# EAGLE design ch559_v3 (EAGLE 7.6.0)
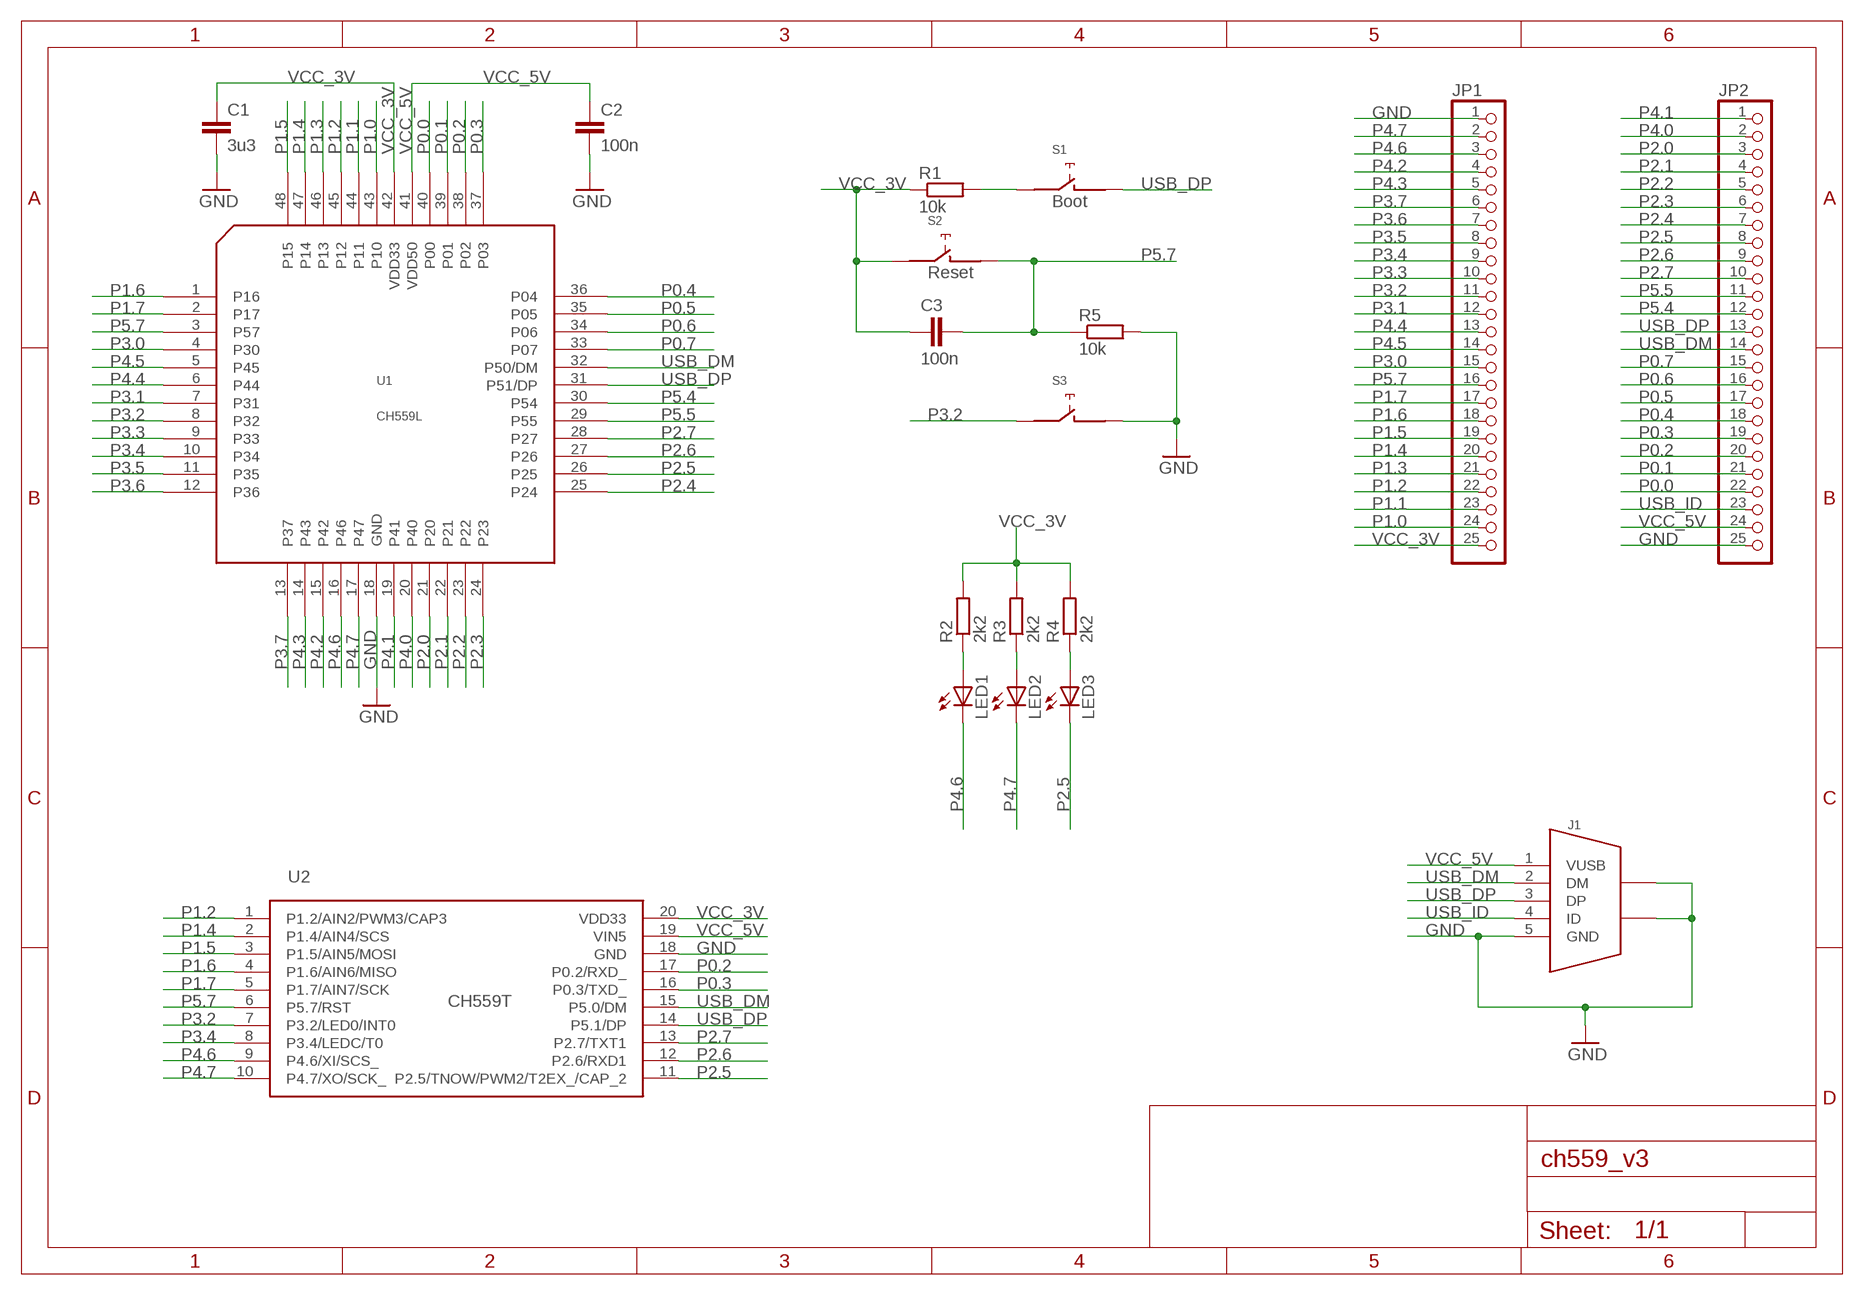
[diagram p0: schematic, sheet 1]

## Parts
C1  3u3  C-EUC0805  [C0805]
C2  100n  C-EUC0805  [C0805]
C3  100n  C-EUC0805  [C0805]
J1  MIC_USB_BBU  [MICRO_USB_B]
JP1  PINHD25  [1X25]
JP2  PINHD25  [1X25]
LED1  LEDSML0805  [SML0805]
LED2  LEDSML0805  [SML0805]
LED3  LEDSML0805  [SML0805]
R1  10k  R-EU_R0603  [R0603]
R2  2k2  R-EU_R0603  [R0603]
R3  2k2  R-EU_R0603  [R0603]
R4  2k2  R-EU_R0603  [R0603]
R5  10k  R-EU_R0603  [R0603]
S1  KMR_231_G_LFS  [KMR_231]
S2  KMR_231_G_LFS  [KMR_231]
S3  KMR_231_G_LFS  [KMR_231]
U1  CH559L  [LQFP48]
U2  CH559T  [SSOP20]

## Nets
GND: C1.2 C2.2 J1.5(GND) J1.P3(SHIELD) J1.P4(SHIELD) JP1.1 JP2.25 R5.2 S3.P$3 S3.P$4 U1.18(GND) U2.18(GND)
N$2: LED1.A R2.1
N$30: R1.2 S1.P$1 S1.P$2
N$43: LED2.A R3.1
N$44: LED3.A R4.1
P0.0: JP2.22 U1.40(P00)
P0.1: JP2.21 U1.39(P01)
P0.2: JP2.20 U1.38(P02) U2.17(P0.2/RXD_)
P0.3: JP2.19 U1.37(P03) U2.16(P0.3/TXD_)
P0.4: JP2.18 U1.36(P04)
P0.5: JP2.17 U1.35(P05)
P0.6: JP2.16 U1.34(P06)
P0.7: JP2.15 U1.33(P07)
P1.0: JP1.24 U1.43(P10)
P1.1: JP1.23 U1.44(P11)
P1.2: JP1.22 U1.45(P12) U2.1(P1.2/AIN2/PWM3/CAP3)
P1.3: JP1.21 U1.46(P13)
P1.4: JP1.20 U1.47(P14) U2.2(P1.4/AIN4/SCS)
P1.5: JP1.19 U1.48(P15) U2.3(P1.5/AIN5/MOSI)
P1.6: JP1.18 U1.1(P16) U2.4(P1.6/AIN6/MISO)
P1.7: JP1.17 U1.2(P17) U2.5(P1.7/AIN7/SCK)
P2.0: JP2.3 U1.21(P20)
P2.1: JP2.4 U1.22(P21)
P2.2: JP2.5 U1.23(P22)
P2.3: JP2.6 U1.24(P23)
P2.4: JP2.7 U1.25(P24)
P2.5: JP2.8 LED3.C U1.26(P25) U2.11(P2.5/TNOW/PWM2/T2EX_/CAP_2)
P2.6: JP2.9 U1.27(P26) U2.12(P2.6/RXD1)
P2.7: JP2.10 U1.28(P27) U2.13(P2.7/TXT1)
P3.0: JP1.15 U1.4(P30)
P3.1: JP1.12 U1.7(P31)
P3.2: JP1.11 S3.P$1 S3.P$2 U1.8(P32) U2.7(P3.2/LED0/INT0)
P3.3: JP1.10 U1.9(P33)
P3.4: JP1.9 U1.10(P34) U2.8(P3.4/LEDC/T0)
P3.5: JP1.8 U1.11(P35)
P3.6: JP1.7 U1.12(P36)
P3.7: JP1.6 U1.13(P37)
P4.0: JP2.2 U1.20(P40)
P4.1: JP2.1 U1.19(P41)
P4.2: JP1.4 U1.15(P42)
P4.3: JP1.5 U1.14(P43)
P4.4: JP1.13 U1.6(P44)
P4.5: JP1.14 U1.5(P45)
P4.6: JP1.3 LED1.C U1.16(P46) U2.9(P4.6/XI/SCS_)
P4.7: JP1.2 LED2.C U1.17(P47) U2.10(P4.7/XO/SCK_)
P5.4: JP2.12 U1.30(P54)
P5.5: JP2.11 U1.29(P55)
P5.7: C3.2 JP1.16 R5.1 S2.P$3 S2.P$4 U1.3(P57) U2.6(P5.7/RST)
USB_DM: J1.2(DM) JP2.14 U1.32(P50/DM) U2.15(P5.0/DM)
USB_DP: J1.3(DP) JP2.13 S1.P$3 S1.P$4 U1.31(P51/DP) U2.14(P5.1/DP)
USB_ID: J1.4(ID) JP2.23
VCC_3V: C1.1 C3.1 JP1.25 R1.1 R2.2 R3.2 R4.2 S2.P$1 S2.P$2 U1.42(VDD33) U2.20(VDD33)
VCC_5V: C2.1 J1.1(VUSB) JP2.24 U1.41(VDD50) U2.19(VIN5)

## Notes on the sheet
- Boot
- Reset

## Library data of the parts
C1-C3 = rcl:C-EU: CAPACITOR, European symbol
J1 = tzlib:MIC_USB_BBU
JP1 JP2 = tzlib:PINHD25
LED1-LED3 = led:LED: LED
R1-R5 = rcl:R-EU_: RESISTOR, European symbol
S1-S3 = tzlib:KMR_231_G_LFS
U1 = tzlib:CH559L
U2 = tzlib:CH559T

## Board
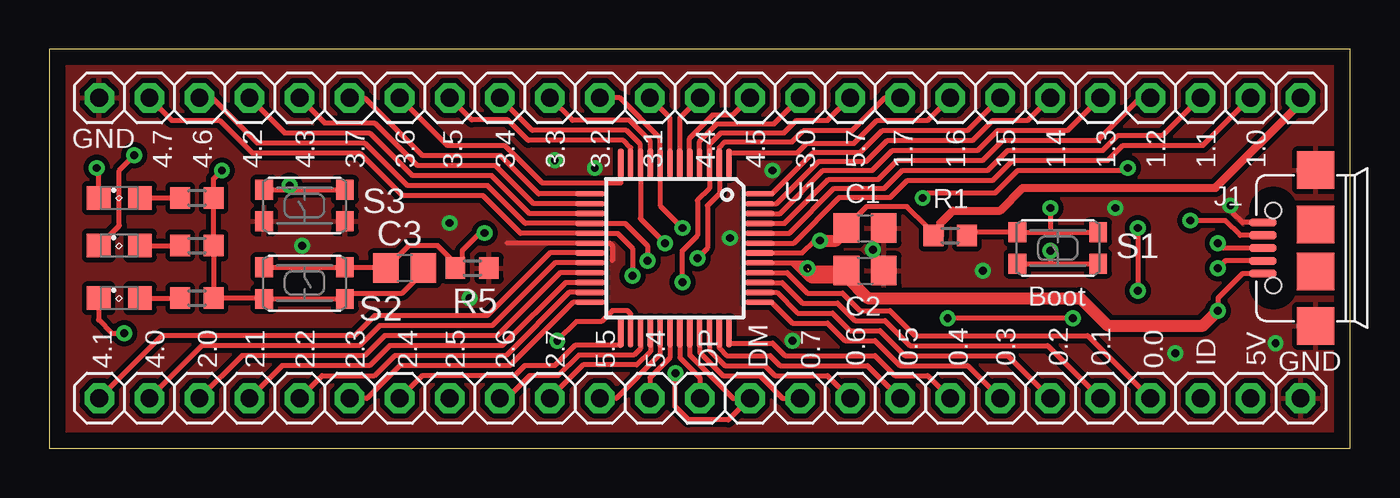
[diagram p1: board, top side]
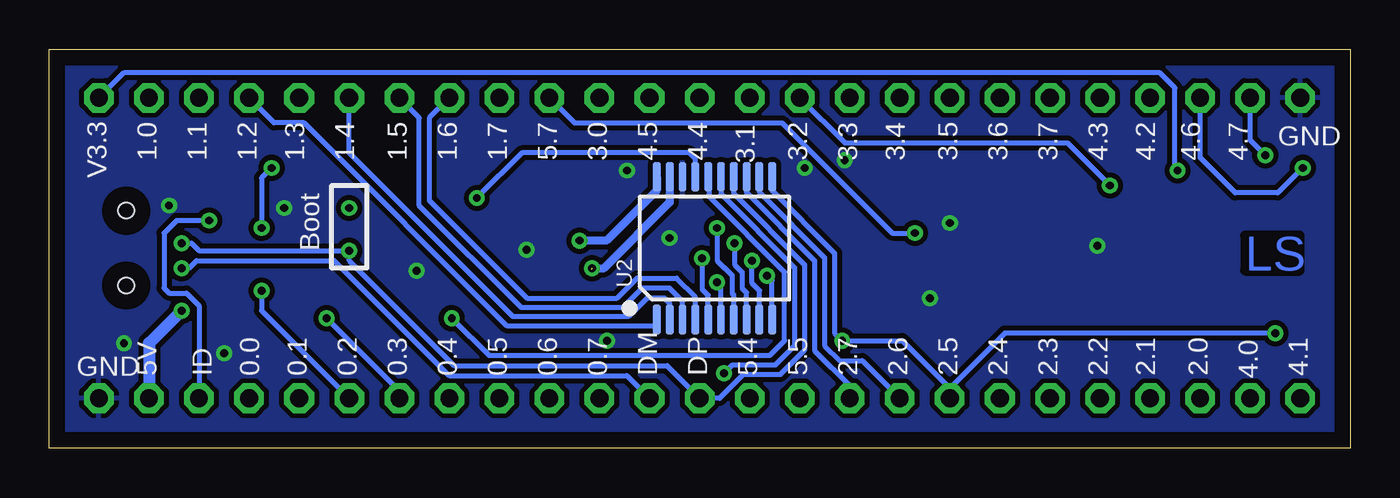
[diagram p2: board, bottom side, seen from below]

Size 66.02 x 20.24 mm. Coordinates in mm from the lower left corner, seen from the top.
Outline: 0,0 66.02,0 66.02,20.24 0,20.24 0,0
Copper layers (1*16): Top 0.035mm / dielectric 1.5mm / Bottom 0.035mm
Design rules "default *": minimum track width 8mil, minimum drill 0.4mm, track to track 0.16mm, track to pad 0.16mm, pad to pad 0.2mm, via to via 0.2mm, smd to smd 0.2mm, copper to edge 32mil, drill to drill 8mil, minimum pad ring 10mil, minimum via ring 8mil, stop-mask expansion 4mil, vias tented up to drill 0mil, thermal gap 10mil

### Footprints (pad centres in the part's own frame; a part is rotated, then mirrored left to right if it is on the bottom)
C0805 = smd 1.3 x 1.5: 1 -0.95,0; 2 0.95,0
MICRO_USB_B = smd 0.4 x 1.4: 1 -1.3,2.675; 2 -0.65,2.675; 3 0,2.675; 4 0.65,2.675; 5 1.3,2.675 | smd 1.9 x 1.9: P1 -1.2,0; P2 1.2,0; P3 3.95,0; P4 -3.95,0 | hole 0.8: -1.9,2.15; 1.9,2.15
1X25 = drill 0.9 pad 1.5 octagon: 1 -29.21,0; 2 -26.67,0; 3 -24.13,0; 4 -21.59,0; 5 -19.05,0; 6 -16.51,0; 7 -13.97,0; 8 -11.43,0; 9 -8.89,0; 10 -6.35,0; 11 -3.81,0; 12 -1.27,0; 13 1.27,0; 14 3.81,0; 15 6.35,0; 16 8.89,0; 17 11.43,0; 18 13.97,0; 19 16.51,0; 20 19.05,0; 21 21.59,0; 22 24.13,0; 23 26.67,0; 24 29.21,0; 25 31.75,0
SML0805 = smd 1.2 x 1.2: A 1.05,0; C -1.05,0
R0603 = smd 1 x 1.1: 1 -0.85,0; 2 0.85,0
KMR_231 = smd 0.9 x 1: P$1 -2.05,0.8; P$2 2.05,0.8; P$3 -2.05,-0.8; P$4 2.05,-0.8
LQFP48 = smd 1.5 x 0.3: 1 -4.3,2.75; 2 -4.3,2.25; 3 -4.3,1.75; 4 -4.3,1.25; 5 -4.3,0.75; 6 -4.3,0.25; 7 -4.3,-0.25; 8 -4.3,-0.75; 9 -4.3,-1.25; 10 -4.3,-1.75; 11 -4.3,-2.25; 12 -4.3,-2.75; 25 4.3,-2.75; 26 4.3,-2.25; 27 4.3,-1.75; 28 4.3,-1.25; 29 4.3,-0.75; 30 4.3,-0.25; 31 4.3,0.25; 32 4.3,0.75; 33 4.3,1.25; 34 4.3,1.75; 35 4.3,2.25; 36 4.3,2.75 | smd 0.3 x 1.5: 13 -2.75,-4.3; 14 -2.25,-4.3; 15 -1.75,-4.3; 16 -1.25,-4.3; 17 -0.75,-4.3; 18 -0.25,-4.3; 19 0.25,-4.3; 20 0.75,-4.3; 21 1.25,-4.3; 22 1.75,-4.3; 23 2.25,-4.3; 24 2.75,-4.3; 37 2.75,4.3; 38 2.25,4.3; 39 1.75,4.3; 40 1.25,4.3; 41 0.75,4.3; 42 0.25,4.3; 43 -0.25,4.3; 44 -0.75,4.3; 45 -1.25,4.3; 46 -1.75,4.3; 47 -2.25,4.3; 48 -2.75,4.3
SSOP20 = smd 0.4 x 1.5: 1 -2.925,-3.625; 2 -2.275,-3.625; 3 -1.625,-3.625; 4 -0.975,-3.625; 5 -0.325,-3.625; 6 0.325,-3.625; 7 0.975,-3.625; 8 1.625,-3.625; 9 2.275,-3.625; 10 2.925,-3.625; 11 2.925,3.625; 12 2.275,3.625; 13 1.625,3.625; 14 0.975,3.625; 15 0.325,3.625; 16 -0.325,3.625; 17 -0.975,3.625; 18 -1.625,3.625; 19 -2.275,3.625; 20 -2.925,3.625

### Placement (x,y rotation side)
C1  41.4,11.18 0 top
C2  41.4,9.02 0 top
C3  18.03,9.14 180 top
J1  64.26,10.16 90 top
JP1  31.75,17.78 0 top
JP2  31.75,2.54 0 top
LED1  3.56,12.7 0 top
LED2  3.56,10.29 0 top
LED3  3.56,7.62 0 top
R1  45.72,10.79 0 top
R2  7.49,12.7 0 top
R3  7.49,10.29 0 top
R4  7.49,7.62 0 top
R5  21.46,9.14 0 top
S1  51.18,10.16 0 top
S2  12.95,8.38 180 top
S3  12.95,12.32 0 top
U1  31.75,10.16 270 top
U2  32.26,10.16 0 bottom

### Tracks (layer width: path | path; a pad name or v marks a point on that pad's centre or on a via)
GND  (via drill 0.4)
  Top 0.254: 27.44,10.41 27.43,10.41 | J1.5 60.55,11.46 60.07,11.94 | 27.44,10.41 23.24,10.41 | 27.44,10.41 28.45,10.41 28.57,10.29 28.57,9.53
  Top 0.813: J1.P4 64.26,6.1 | J1.P3 64.26,14.61
  other vias: 34.54,10.67 12.83,10.29 20.32,11.43 41.81,10.08 47.37,9.02 57.15,4.83 54.1,12.19 59.94,12.32 62.23,5.33 37.72,5.46 21.34,7.62 27.69,14.22 25.65,14.61 36.7,14.1
  pour Bottom (isolate 0.254): 0.51,20.07 65.79,20.07 65.79,0.13 0.51,0.13
  pour Top (isolate 0.254): 0.25,20.19 66.04,20.19 66.04,0 0.25,0
N$2
  Top 0.254: LED1.A R2.1
N$30  (via drill 0.4)
  Top 0.254: 50.8,10.96 S1.P$1 46.73,10.96 R1.2 | 50.8,10.96 S1.P$2 | v50.8,12.19 50.8,10.96
N$43
  Top 0.254: LED2.A R3.1
N$44
  Top 0.254: LED3.A R4.1
P0.0
  Top 0.254: U1.40 37.45,8.91 38.35,8 38.48,7.87 40.26,7.87 41.15,6.99 42.67,6.99 43.94,5.71 52.7,5.71 JP2.22
P0.1
  Top 0.254: U1.39 37.18,8.41 38.23,7.37 40.01,7.37 40.89,6.48 42.42,6.48 43.69,5.21 50.67,5.21 JP2.21
P0.2  (via drill 0.4)
  Top 0.254: U1.38 36.92,7.91 37.97,6.86 39.75,6.86 40.64,5.97 42.16,5.97 43.43,4.7 48.64,4.7 JP2.20 | v44.32,12.7 44.58,12.95 48.01,12.95 49.15,14.1 54.61,14.1 v54.74,14.22 | v55.25,11.18 v55.25,8
  Bottom 0.254: v54.74,14.22 55.25,13.72 v55.25,11.18 | JP2.20 55.25,6.99 v55.25,8 | U2.17 33.23,14.69 33.53,14.99 42.04,14.99 v44.32,12.7
P0.3  (via drill 0.4)
  Top 0.254: U1.37 36.66,7.41 37.72,6.35 39.5,6.35 40.39,5.46 41.91,5.46 43.18,4.19 46.61,4.19 JP2.19 | v51.94,6.6 v45.59,6.6
  Bottom 0.254: JP2.19 48.26,2.92 v51.94,6.6 | v45.59,6.6 43.69,4.7 29.46,4.7 28.7,5.46 28.7,8.94 32.51,12.75 32.51,13.71 U2.16
P0.4
  Top 0.254: U1.36 34.5,5.38 34.54,5.33 36.7,5.33 37.34,4.7 41.91,4.7 42.93,3.68 44.58,3.68 JP2.18
P0.5
  Top 0.254: U1.35 34,5.08 34.38,4.7 36.58,4.7 37.08,4.19 41.53,4.19 JP2.17
P0.6
  Top 0.254: JP2.16 39.5,3.68 36.83,3.68 36.32,4.19 34.29,4.19 33.5,4.98 U1.34
P0.7
  Top 0.254: U1.33 33,4.87 34.19,3.68 36.07,3.68 37.21,2.54 JP2.15
P1.0
  Top 0.254: U1.43 37.78,10.41 40.09,12.72 42.7,12.72 43.56,13.59 47.88,13.59 48.89,14.61 53.72,14.61 54.48,15.37 58.55,15.37 JP1.24
P1.1
  Top 0.254: U1.44 37.55,10.91 39.83,13.18 42.39,13.18 43.31,14.1 47.62,14.1 48.64,15.11 53.47,15.11 54.23,15.88 56.52,15.88 JP1.23
P1.2
  Top 0.254: U1.45 37.32,11.41 39.55,13.64 42.09,13.64 43.05,14.61 47.37,14.61 48.39,15.62 53.21,15.62 55.37,17.78 JP1.22
  Bottom 0.254: JP1.22 54.61,16.51 53.09,16.51 42.78,6.2 35.35,6.2 35.18,6.37 U2.1
P1.3
  Top 0.254: U1.46 37.08,11.91 39.27,14.1 41.78,14.1 42.8,15.11 47.12,15.11 48.13,16.13 51.69,16.13 JP1.21
P1.4
  Top 0.254: U1.47 36.91,12.41 39.05,14.55 41.48,14.55 42.55,15.62 46.86,15.62 47.88,16.64 49.66,16.64 JP1.20
  Bottom 0.254: JP1.20 50.8,14.99 42.49,6.68 36.63,6.68 35.69,7.62 34.8,7.62 34.53,7.36 U2.2
P1.5
  Top 0.254: JP1.19 46.61,16.13 42.29,16.13 41.17,15.01 38.79,15.01 36.68,12.91 U1.48
  Bottom 0.254: JP1.19 47.24,16.76 47.24,12.32 42.06,7.14 36.93,7.14 35.94,8.13 34.54,8.13 33.88,7.47 U2.3
P1.6
  Top 0.254: JP1.18 44.58,16.64 42.01,16.64 40.84,15.47 38.46,15.47 37.97,14.99 34.52,14.99 34.5,14.97 U1.1
  Bottom 0.254: JP1.18 46.74,16.76 46.74,12.57 41.78,7.62 37.21,7.62 36.2,8.64 34.19,8.64 33.23,7.68 U2.4
P1.7  (via drill 0.4)
  Top 0.254: v32.89,9.65 33.4,10.16 33.4,12.32 34,12.92 U1.2 34,15.25 34.29,15.54 37.69,15.54 38.25,16.1 40.74,16.1 42.42,17.78 JP1.17
  Bottom 0.254: U2.5 32.58,7.77 32.89,8.08 v32.89,9.65
P2.0
  Top 0.254: U1.21 25.93,8.91 22.73,5.71 17.02,5.71 16,4.7 9.78,4.7 JP2.3
P2.1
  Top 0.254: U1.22 26.19,8.41 22.99,5.21 17.27,5.21 16.26,4.19 11.81,4.19 JP2.4
P2.2
  Top 0.254: U1.23 26.39,7.91 23.18,4.7 17.53,4.7 16.51,3.68 13.84,3.68 JP2.5
P2.3
  Top 0.254: U1.24 26.59,7.41 23.37,4.19 17.78,4.19 16.13,2.54 JP2.6
P2.4
  Top 0.254: U1.25 29,5.25 28.97,5.23 26.69,5.23 25.65,4.19 24.13,4.19 23.62,3.68 18.92,3.68 JP2.7
P2.5  (via drill 0.4)
  Top 0.254: U1.26 29.5,6.82 29.34,6.99 28.57,6.99 28.02,6.43 26.75,6.43 v25.78,5.46 | LED3.C 2.51,6.51 3.18,5.84 v3.81,5.84
  Bottom 0.254: 20.32,3.05 22.73,5.46 v25.78,5.46 26.16,5.84 26.16,9.91 29.34,13.08 U2.11 | 20.32,3.05 JP2.8 | v3.81,5.84 17.53,5.84 20.32,3.05
P2.6
  Top 0.254: U1.27 30,5.06 29.67,4.72 26.87,4.72 25.83,3.68 24.38,3.68 23.24,2.54 JP2.9
  Bottom 0.254: JP2.9 24.77,4.45 25.91,4.45 26.67,5.21 26.67,9.68 29.97,12.98 U2.12
P2.7
  Top 0.254: U1.28 30.5,4.91 29.82,4.23 27.09,4.23 JP2.10
  Bottom 0.254: JP2.10 25.4,3.17 27.18,4.95 27.18,9.53 30.63,12.98 U2.13
P3.0
  Top 0.254: U1.4 33,15.58 33.88,16.46 36.78,16.46 JP1.15
P3.1
  Top 0.254: U1.7 31.5,16.76 JP1.12
P3.2  (via drill 0.4)
  Top 0.254: JP1.11 28.96,17.78 31,15.74 U1.8 31,12.31 v32.13,11.18 | v12.19,13.34 12.15,13.34 12.19,13.12 | S3.P$1 12.19,13.12 | 12.19,13.12 S3.P$2
  Bottom 0.254: 12.19,13.59 v12.19,13.34 14.35,15.49 25.65,15.49 JP1.11 | v32.13,11.18 32.13,9.53 31.75,9.14 31.75,9.17 31.37,8.79 31.37,7.87 31.29,7.8 31.29,7.77 31.28,7.76 U2.7
P3.3
  Top 0.254: U1.9 30.5,15.58 29.44,16.64 26.54,16.64 JP1.10
P3.4  (via drill 0.4)
  Top 0.254: JP1.9 24.51,16.13 29.29,16.13 30,15.41 U1.10 30,11.66 v31.24,10.41
  Bottom 0.254: v31.24,10.41 31.24,9.32 30.86,8.94 30.86,8.13 30.63,7.9 U2.8 30.61,6.56
P3.5
  Top 0.254: U1.11 29.5,15.25 29.13,15.62 24.31,15.62 23.27,16.66 21.44,16.66 JP1.8
P3.6
  Top 0.254: 29,14.94 U1.12 29,13.46 25.02,13.46 23.11,15.37 20.19,15.37 JP1.7
P3.7
  Top 0.254: U1.13 24.83,12.91 22.88,14.86 18.92,14.86 16,17.78 JP1.6
P4.0
  Top 0.254: U1.20 25.67,9.41 22.48,6.22 16.76,6.22 15.75,5.21 7.75,5.21 JP2.2
P4.1
  Top 0.254: U1.19 25.4,9.91 22.23,6.73 16.51,6.73 15.49,5.71 5.71,5.71 JP2.1
P4.2
  Top 0.254: U1.15 24.36,11.91 22.43,13.84 18.41,13.84 16.26,16 11.94,16 JP1.4
P4.3
  Top 0.254: U1.14 24.57,12.41 22.63,14.35 18.67,14.35 16.51,16.51 13.97,16.51 JP1.5
P4.4
  Top 0.254: U1.6 32,16.76 JP1.13
P4.5
  Top 0.254: U1.5 32.5,15.74 33.68,16.92 34.7,16.92 JP1.14
P4.6  (via drill 0.4)
  Top 0.254: JP1.3 8.25,17.78 10.54,15.49 16,15.49 18.16,13.34 22.23,13.34 24.15,11.41 U1.16 29.23,11.41 30.35,10.29 v30.35,9.53 | LED1.C 2.51,14.13 v2.41,14.22
  Bottom 0.254: v2.41,14.22 3.68,12.95 5.84,12.95 7.62,14.73 JP1.3 | U2.9 29.98,7.25 29.97,7.26 29.97,8 30.35,8.38 v30.35,9.53
P4.7  (via drill 0.4)
  Top 0.254: JP1.2 6.22,16.64 8.64,16.64 10.29,14.99 15.75,14.99 17.91,12.83 22,12.83 23.91,10.91 U1.17 28.84,10.91 29.59,10.16 v29.59,8.76 | LED2.C 2.54,10.29 3.56,11.3 3.56,14.1 v4.32,14.86
  Bottom 0.254: v4.32,14.86 5.08,15.62 JP1.2 | U2.10 29.33,8.51 v29.59,8.76
P5.4
  Top 0.254: U1.30 31.5,4.6 30.48,3.58 JP2.12
P5.5
  Top 0.254: U1.29 31,4.76 28.78,2.54 JP2.11 28.3,2.54
P5.7  (via drill 0.4)
  Top 0.254: v32.13,8.43 32.13,10.03 32.89,10.79 32.89,12.57 33.5,13.18 U1.3 33.5,15.41 34.09,16 37.29,16 37.92,16.64 39.5,16.64 JP1.16 | S2.P$4 S2.P$3 17.08,9.18 C3.2 18.23,10.29 19.71,10.29 20.34,9.65 20.34,9.41 R5.1 | R5.1 20.61,9.36 | R5.1 20.95,9.49 20.95,10.03 21.84,10.92 v22.1,10.92
  Bottom 0.254: JP1.16 39.37,16.51 28.83,16.51 23.24,10.92 v22.1,10.92 | U2.6 31.93,8.23 v32.13,8.43
USB_DM  (via drill 0.4, 0.4 pad 0.8)
  Top 0.254: U1.32 32.5,4.74 34.7,2.54 JP2.14 34.47,1.45 32.44,1.45 31.75,2.13 31.75,3.78 v31.77,3.8 | J1.2 59.67,9.51 v59.31,9.14
  Bottom 0.254: v59.31,9.14 58.93,9.14 58.55,9.53 51.56,9.53 45.72,3.68 36.7,3.68 JP2.14 | U2.15 31.9,13.75 31.9,12.88 28.19,9.17 28.19,5.21 29.18,4.22 31.36,4.22 v31.77,3.8 31.69,3.8
USB_DP  (via drill 0.4)
  Top 0.254: U1.31 32,4.6 33.02,3.58 JP2.13 | J1.3 59.56,10.16 v59.31,10.41 | S1.P$3 50.8,9.36 | 50.8,9.36 S1.P$4 | v50.8,10.03 50.8,9.36
  Bottom 0.254: v59.31,10.41 58.8,10.41 58.42,10.03 v50.8,10.03 50.8,9.53 45.47,4.19 34.67,4.19 JP2.13 32,2.54 30.81,3.73 28.93,3.73 27.69,4.98 27.69,9.32 31.27,12.9 31.27,13.77 U2.14
USB_ID  (via drill 0.4)
  Top 0.254: J1.4 60.44,10.81 59.69,11.56 v57.91,11.56
  Bottom 0.254: v57.91,11.56 59.56,11.56 60.2,10.92 60.2,8.13 59.94,7.87 59.05,7.87 58.42,7.24 JP2.23
VCC_3V  (via drill 0.4)
  Top 0.254: 44.87,10.88 R1.1 44.53,11.14 44.53,11.28 43.54,12.27 41.48,12.27 40.64,11.43 40.64,10.99 | R3.2 R4.2 10.92,7.62 10.92,7.58 S2.P$2 S2.P$1 15.07,7.58 15.37,7.87 17.91,7.87 18.54,8.51 18.54,8.7 C3.1 | R3.2 8.25,10.29 | R3.2 R2.2 8.34,13.68 v8.76,14.1 | U1.42 38.21,9.91 38.84,10.54 v39.12,10.54 | 39.94,10.54 39.94,10.67 C1.1 40.64,10.99 | 40.64,10.98 40.64,10.99
  Top 0.406: 44.87,10.88 44.96,10.79 45.21,10.79 45.21,11.43 45.85,12.06 48.26,12.06 49.4,13.21 59.18,13.21 63.5,17.53 JP1.25
  Top 0.61: v39.12,10.54 39.94,10.54
  Bottom 0.254: v8.76,14.1 8.89,14.22 8.89,18.29 9.65,19.05 62.23,19.05 JP1.25
  Bottom 0.406: U2.20 35.18,13.1 37.74,10.54 v39.12,10.54
VCC_5V  (via drill 0.4)  (1 unrouted)
  Top 0.254: U1.41 38.47,9.41 38.61,9.27 38.61,9.25 arc-45 38.53,9.07 38.48,9.02 | 37.72,9.4 38.23,8.89 | 38.23,8.89 38.23,9.27 38.1,9.27 | J1.1 60.55,8.86 59.31,7.62 v59.31,6.99 | 40.34,9.14 v38.48,9.14 38.23,8.89
  Top 0.61: C2.1 40.45,8.7 41.53,7.62 52.32,7.62 53.72,6.22 58.55,6.22 v59.31,6.99
  Top 0.813: C2.1 40.39,9.02 40.39,8.76 38.73,8.76 38.48,9.02
  Bottom 0.254: 38.61,9.14 v38.48,9.14
  Bottom 0.406: U2.19 34.53,12.48 37.9,9.12 38.46,9.12 v38.48,9.14
  Bottom 0.61: v59.31,6.99 60.96,5.33 JP2.24

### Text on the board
Bottom: LS
tPlace: GND | 4.7 | 4.6 | 4.2 | 4.3 | 3.7 | 3.6 | 3.5 | 3.4 | 3.3 | 3.2 | 3.1 | 4.4 | 4.5 | 3.0 | 5.7 | 1.7 | 1.6 | 1.5 | 1.4 | 1.3 | 1.2 | 1.1 | 1.0 | Boot | 4.1 | 4.0 | 2.0 | 2.1 | 2.2 | 2.3 | 2.4 | 2.5 | 2.6 | 2.7 | 5.5 | 5.4 | DP | DM | 0.7 | 0.6 | 0.5 | 0.4 | 0.3 | 0.2 | 0.1 | 0.0 | ID | 5V | GND
bPlace: GND | 4.7 | 4.6 | 4.2 | 4.3 | 3.7 | 3.6 | 3.5 | 3.4 | 3.3 | 3.2 | 3.1 | 4.4 | 4.5 | 3.0 | 5.7 | 1.7 | 1.6 | 1.5 | 1.4 | 1.3 | 1.2 | 1.1 | 1.0 | V3.3 | Boot | 4.1 | 2.0 | 2.1 | 2.2 | 2.3 | 2.4 | 2.5 | 2.6 | 2.7 | 5.5 | 5.4 | DP | DM | 0.7 | 0.6 | 0.5 | 0.4 | 0.3 | 0.2 | 0.1 | 0.0 | ID | 5V | GND | 4.0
